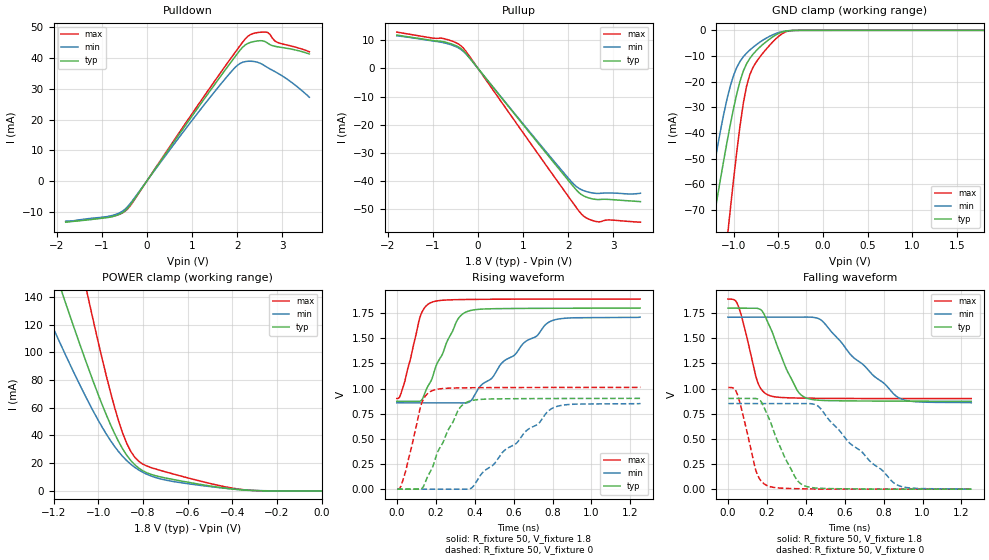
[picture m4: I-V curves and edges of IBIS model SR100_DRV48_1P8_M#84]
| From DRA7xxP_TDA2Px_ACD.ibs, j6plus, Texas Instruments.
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| Model based on original model for DDR_SEIOPB_V
|   Sub model SR100_DRV48_1P8
[model]   SR100_DRV48_1P8_M#84
|[Description]  [1.8V-I/O-X-X]
|   , ,
|[Input Load]
|[Output Drive]
|Voltage   1.8V
|Mode   I/O
Model_type   I/O
Polarity   Non-Inverting
Enable   Active-Low
Vinl =  0.775
Vinh =  1.025
Cref =  15.0000pF
Rref =  100.0000M
Vref =  0V
Vmeas =  0.9
C_comp   2p   2p   2p
[Model Spec]
Vinl   0.78   0.735   0.825
Vinh   1.02   0.975   1.065
[Receiver Thresholds]
Tslew_ac = 0.5n
Vth = 0.9
Vth_max = 0.945
Vth_min = 0.81
Vinh_ac = 0.2
Vinh_dc = 0.125
Vinl_ac = -0.2
Vinl_dc = -0.125
[Temperature Range]   25   125   -40
[Voltage Range]   1.8   1.71   1.89
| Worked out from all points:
|   slope of the pulldown table from 0 to 0.27 V, typ, clamps not added: 46.9 ohm
|   slope of the pullup table from 0 to 0.27 V, typ, clamps not added: 49.7 ohm
|   GND clamp passes 1 mA (typ) near -0.48 V on its own axis
|   POWER clamp passes 1 mA (typ) near -0.38 V on its own axis
|   rising waveform, R_fixture 50, V_fixture 1.8: 20-80 % time 125ps typ, 296ps min, 71.8ps max; typ from 0.874 V to 1.8 V
|   rising waveform, R_fixture 50, V_fixture 0: 20-80 % time 126ps typ, 297ps min, 71.8ps max; typ from 0 V to 0.903 V
|   falling waveform, R_fixture 50, V_fixture 1.8: 20-80 % time 119ps typ, 271ps min, 73.2ps max; typ from 1.8 V to 0.874 V
|   falling waveform, R_fixture 50, V_fixture 0: 20-80 % time 123ps typ, 279ps min, 72.8ps max; typ from 0.903 V to 0 V
[POWER_clamp]
-1.8V     464.6mA    344.4mA    740.8mA
-1.273V   197mA      143.3mA    314.4mA
-1.164V   144mA      104.2mA    229mA
-1.145V   135.3mA    97.86mA    215mA
-1.055V   93.25mA    67.59mA    146.5mA
-1.036V   85.18mA    61.89mA    133.3mA
-909.1mV  35.72mA    28.41mA    50.73mA
-872.7mV  25.87mA    21.94mA    34.5mA
-818.2mV  16.45mA    15.08mA    21.33mA
-690.9mV  9.084mA    7.592mA    13.42mA
-400mV    1.38mA     1.43mA     2.039mA
0V        227.3nA    761nA      1.176uA
[Pulldown]
-1.8V     -13.45mA   -13.11mA   -13.3mA
-818.2mV  -11.81mA   -11.44mA   -11.72mA
-600mV    -10.83mA   -10.36mA   -10.81mA
-436.4mV  -9.068mA   -8.512mA   -9.288mA
1.255V    26.38mA    24.53mA    27.32mA
1.855V    38.53mA    35.35mA    39.84mA
2.073V    42.76mA    38.34mA    44.25mA
2.291V    45.11mA    39mA       47.65mA
2.618V    45.4mA     37.45mA    48.49mA
2.727V    44.4mA     36.48mA    47.76mA
2.891V    43.71mA    35.16mA    45.15mA
3.6V      41.36mA    27.26mA    42.08mA
[Pullup]
-1.8V     11.9mA     11.66mA    12.97mA
-1.036V   10.04mA    9.888mA    10.91mA
-763.6mV  9.523mA    9.186mA    10.68mA
-490.9mV  8.144mA    7.787mA    9.204mA
-327.3mV  6.377mA    6.133mA    7.311mA
2.018V    -40.23mA   -39.43mA   -46mA
2.182V    -43.37mA   -42.12mA   -49.65mA
2.345V    -45.48mA   -43.6mA    -52.72mA
2.509V    -46.4mA    -44.3mA    -54.07mA
2.673V    -46.74mA   -44.55mA   -54.7mA
2.891V    -46.69mA   -44.38mA   -54.01mA
3.6V      -47.48mA   -44.49mA   -54.81mA
[GND_clamp]
-1.8V     -200.8mA   -187.9mA   -345.9mA
-1.327V   -95.75mA   -76.22mA   -171.1mA
-1.255V   -80.19mA   -60.47mA   -144.9mA
-1.218V   -72.53mA   -52.92mA   -131.9mA
-1.073V   -43.32mA   -26.59mA   -81.54mA
-1.036V   -36.61mA   -21.6mA    -69.55mA
-963.6mV  -24.61mA   -14.37mA   -47.01mA
-854.5mV  -12.98mA   -8.864mA   -21.66mA
-781.8mV  -9.263mA   -6.573mA   -14.36mA
-672.7mV  -5.498mA   -3.827mA   -8.897mA
-345.5mV  -48.81uA   -73.08uA   -79.37uA
1.8V      227.3nA    3.986uA    988nA
[Ramp]
dV/dt_f 0.55612896/0.1195479n 0.51151814/0.27088698n 0.59378876/73.274496p
dV/dt_r 0.54245217/0.12617471n 0.51214857/0.29754451n 0.60767507/71.931913p
R_load = 50
[Rising Waveform]
R_fixture = 50
V_fixture = 1.8
V_fixture_min = 1.71
V_fixture_max = 1.89
0s        873.8mV    858.6mV    901.6mV
16.01ps   873.8mV    858.6mV    922.9mV
39.08ps   873.2mV    858.6mV    1.058V
122ps     877.1mV    858.6mV    1.726V
177.8ps   1.084V     858.6mV    1.857V
307.9ps   1.671V     858.4mV    1.884V
365.6ps   1.769V     861.1mV    1.886V
542.8ps   1.795V     1.261V     1.889V
786.8ps   1.798V     1.666V     1.89V
1.25ns    1.8V       1.71V      1.89V
[Rising Waveform]
R_fixture = 50
V_fixture = 0
V_fixture_min = 0
V_fixture_max = 0
1.768ps   0V         0V         0V
19.19ps   0V         0V         22.74mV
42.34ps   0V         0V         155.9mV
127ps     4.899mV    0V         850mV
183.5ps   216.6mV    0V         980.8mV
313.5ps   778.9mV    0V         1.006V
371.3ps   873.7mV    0V         1.008V
549ps     898.7mV    378mV      1.01V
800.7ps   901.3mV    805.9mV    1.011V
1.252ns   902.5mV    851.6mV    1.011V
[Falling Waveform]
R_fixture = 50
V_fixture = 1.8
V_fixture_min = 1.71
V_fixture_max = 1.89
0s        1.8V       1.71V      1.89V
50.16ps   1.8V       1.71V      1.836V
150.5ps   1.798V     1.71V      1.077V
208.9ps   1.644V     1.71V      934.6mV
346.5ps   1.016V     1.71V      906.5mV
401.9ps   907.4mV    1.711V     904.7mV
484.4ps   882.5mV    1.673V     903.1mV
636.3ps   877.4mV    1.325V     901.6mV
879.3ps   875.1mV    907.1mV    900.9mV
1.25ns    873.8mV    858.6mV    900.8mV
[Falling Waveform]
R_fixture = 50
V_fixture = 0
V_fixture_min = 0
V_fixture_max = 0
1.768ps   902.5mV    851.6mV    1.011V
45.24ps   902.7mV    851.6mV    958.2mV
144.8ps   901.3mV    851.6mV    179.8mV
202.9ps   738.3mV    851.6mV    34.14mV
298.7ps   289.5mV    851.5mV    7.545mV
396.2ps   31.58mV    851.9mV    3.153mV
467.1ps   9.193mV    819.5mV    0V
621.2ps   3.149mV    465.6mV    0V
866.9ps   0V         44.82mV    0V
1.252ns   0V         0V         0V
